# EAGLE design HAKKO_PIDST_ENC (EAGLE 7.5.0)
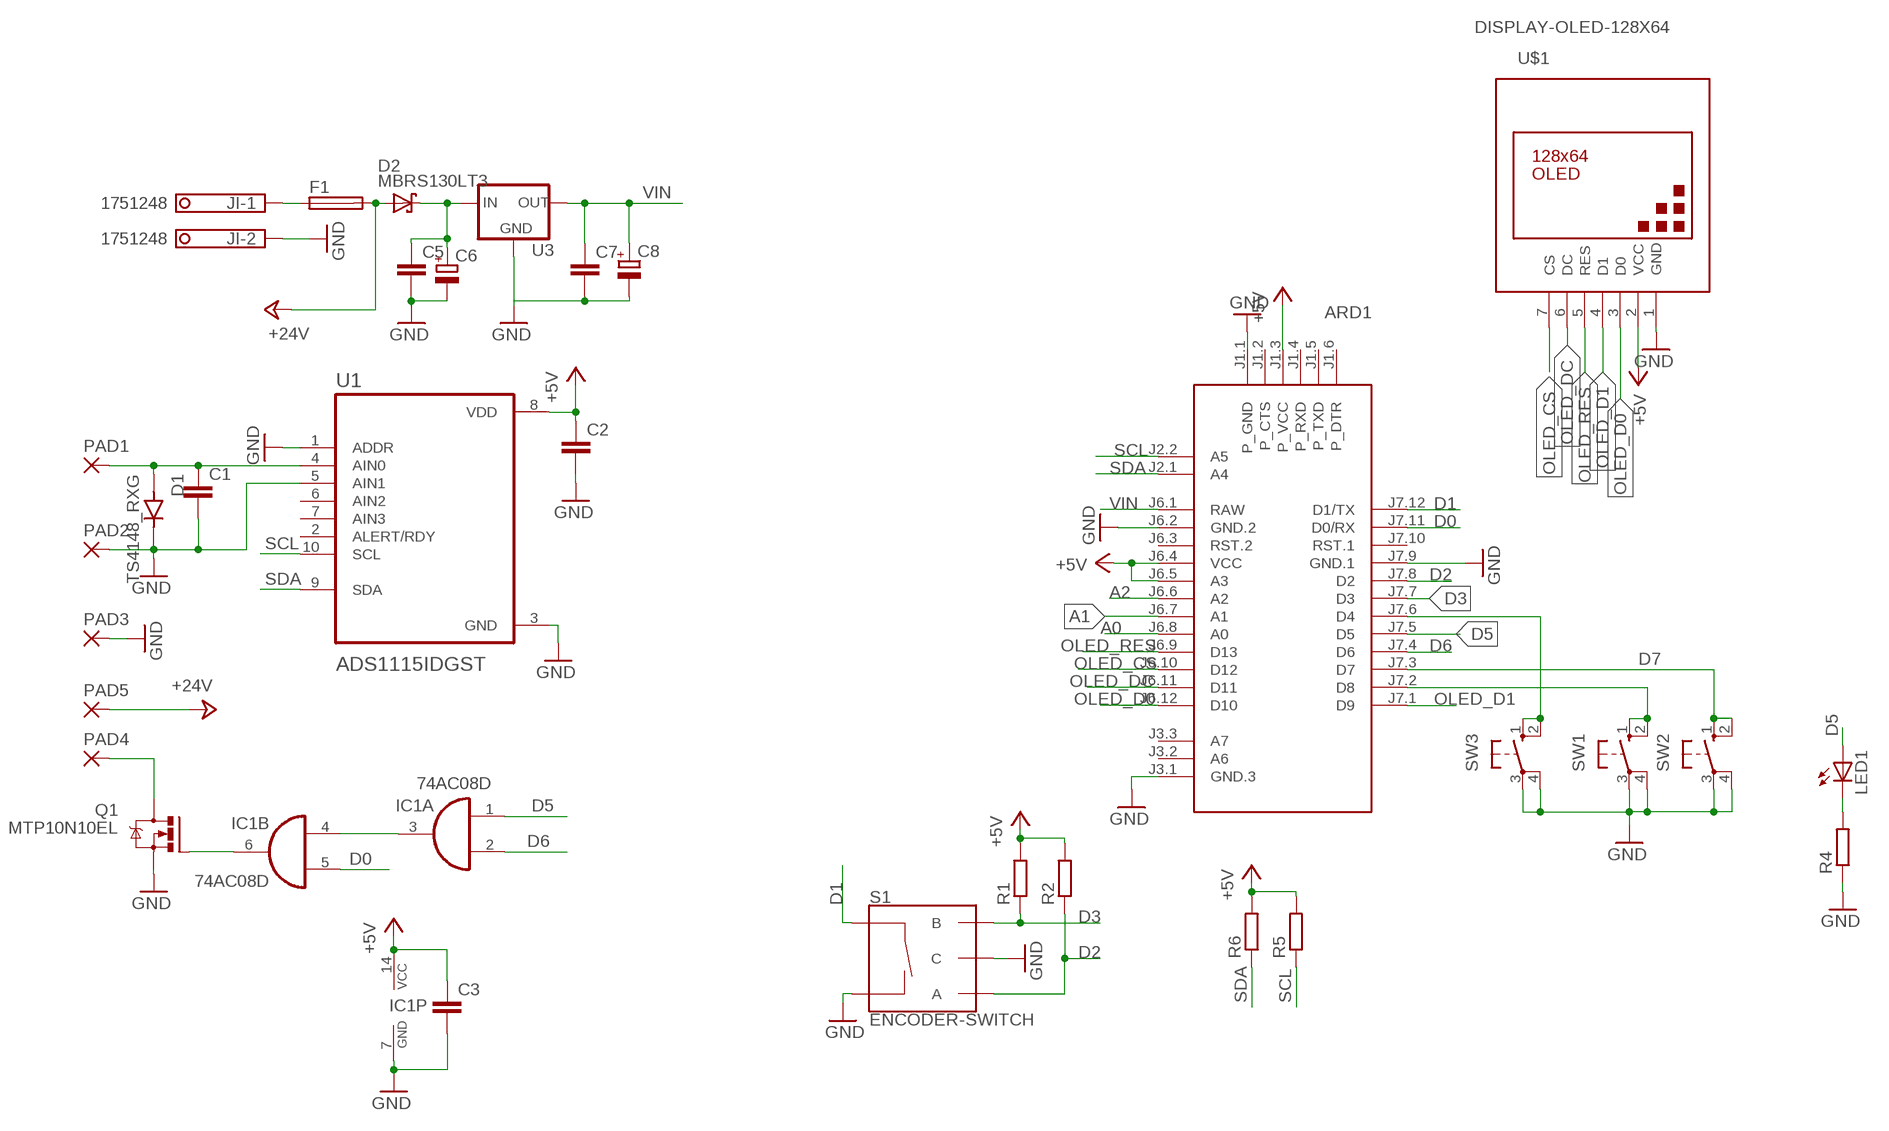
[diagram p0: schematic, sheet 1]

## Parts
ARD1  ARDUINO-PRO-MINI-3.3V  [ARDUINO-PRO-MINI]
C1  C-EUC1206  [C1206]
C2  C-EUC1206  [C1206]
C3  C-EUC1206  [C1206]
C5  C-EUC1206  [C1206]
C6  CPOL-EUSMCB  [SMC_B]
C7  C-EUC1206  [C1206]
C8  CPOL-EUSMCB  [SMC_B]
D1  TS4148_RXG  [DIO_TS4148_RXG]
D2  MBRS130LT3  [SMB]
F1  SH22,5  [SH22,5]
IC1  74AC08D  [SO14]
JI  1751248  [1751248]
LED1  LED5MM  [LED5MM]
PAD1  2,15/1,0  [2,15/1,0]
PAD2  2,15/1,0  [2,15/1,0]
PAD3  2,15/1,0  [2,15/1,0]
PAD4  2,15/1,0  [2,15/1,0]
PAD5  2,15/1,0  [2,15/1,0]
Q1  MTP10N10EL  IRLZ44Z  [TO220BH]
R1  R-EU_R1206  [R1206]
R2  R-EU_R1206  [R1206]
R4  R-EU_R1206  [R1206]
R5  R-EU_R1206  [R1206]
R6  R-EU_R1206  [R1206]
S1  ENCODER-SWITCH  [ROTARY_ENC_PLAIN]
SW1  10-XX  [B3F-10XX]
SW2  10-XX  [B3F-10XX]
SW3  10-XX  [B3F-10XX]
U1  ADS1115IDGST  [SOP50P490X110-10N]
U3  78LXX  [78LXX]
U$1  DISPLAY-OLED-128X64  [DISPLAY-OLED-128X64]

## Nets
+5V: ARD1.J1.3(P_VCC) ARD1.J6.4(VCC) ARD1.J6.5(A3) C2.1 C3.1 IC1.14(P:VCC) R1.2 R2.2 R5.2 R6.2 U1.8(VDD) U$1.2(VCC)
+24V: D2.A F1.2 PAD5.1(P)
A0: ARD1.J6.8(A0)
A1: ARD1.J6.7(A1)
A2: ARD1.J6.6(A2)
D0: ARD1.J7.11(D0/RX) IC1.5(B:I1)
D1: ARD1.J7.12(D1/TX) S1.SW+
D2: ARD1.J7.8(D2) R2.1 S1.A
D3: ARD1.J7.7(D3) R1.1 S1.B
D5: ARD1.J7.5(D5) IC1.1(A:I0) LED1.A
D6: ARD1.J7.4(D6) IC1.2(A:I1)
D7: ARD1.J7.3(D7) SW2.1(S) SW2.2(S1)
GND: ARD1.J1.1(P_GND) ARD1.J3.1(GND.3) ARD1.J6.2(GND.2) ARD1.J7.9(GND.1) C1.2 C2.2 C3.2 C5.2 C6.- C7.2 C8.- D1.C(K) IC1.7(P:GND) JI.2 PAD2.1(P) PAD3.1(P) Q1.S R4.1 S1.C S1.SW- SW1.3(P) SW1.4(P1) SW2.3(P) SW2.4(P1) SW3.3(P) SW3.4(P1) U1.1(ADDR) U1.3(GND) U1.5(AIN1) U3.GND U$1.1(GND)
N$1: C1.1 D1.A PAD1.1(P) U1.4(AIN0)
N$2: PAD4.1(P) Q1.D
N$3: IC1.3(A:O) IC1.4(B:I0)
N$4: F1.1 JI.1
N$6: C5.1 C6.+ D2.C U3.IN
N$7: LED1.K(C) R4.2
N$8: ARD1.J7.2(D8) SW1.1(S) SW1.2(S1)
N$9: IC1.6(B:O) Q1.G
N$10: ARD1.J7.6(D4) SW3.1(S) SW3.2(S1)
OLED_CS: ARD1.J6.10(D12) U$1.7(CS)
OLED_D0: ARD1.J6.12(D10) U$1.3(D0)
OLED_D1: ARD1.J7.1(D9) U$1.4(D1)
OLED_DC: ARD1.J6.11(D11) U$1.6(DC)
OLED_RES: ARD1.J6.9(D13) U$1.5(RES)
SCL: ARD1.J2.2(A5) R5.1 U1.10(SCL)
SDA: ARD1.J2.1(A4) R6.1 U1.9(SDA)
VIN: ARD1.J6.1(RAW) C7.1 C8.+ U3.OUT
Unconnected: ARD1.J1.2(P_CTS) ARD1.J1.4(P_RXD) ARD1.J1.5(P_TXD) ARD1.J1.6(P_DTR) ARD1.J3.2(A6) ARD1.J3.3(A7) ARD1.J6.3(RST.2) ARD1.J7.10(RST.1) IC1.8(C:O) IC1.9(C:I0) IC1.10(C:I1) IC1.11(D:O) IC1.12(D:I0) IC1.13(D:I1) U1.2(ALERT/RDY) U1.6(AIN2) U1.7(AIN3)

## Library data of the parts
ARD1 = diy-modules:ARDUINO-PRO-MINI-*: Arduino Pro Mini and compatible devices More details available here: https://www.arduino.cc/en/Main/ArduinoBoardProMini Click here to find device on ebay.com
C1-C3 C5 C7 = rcl:C-EU: CAPACITOR, European symbol
C6 C8 = rcl:CPOL-EU: POLARIZED CAPACITOR, European symbol
D1 = TS4148_RXG:TS4148_RXG: Check availability Check availability Check availability; AVAILABILITY: In Stock; CHECK_PRICES: https://www.snapeda.com/parts/TS4148%20RXG/Taiwan+Semiconductor/view-part/?ref=eda; DESCRIPTION: 1206 (Ceramics) 75V 0.15A Switching Diode & Array; MF: Taiwan Semiconductor; MP: TS4148 RXG; PACKAGE: 1206-2 Taiwan Semiconductor; PRICE: None; SNAPEDA_LINK: https://www.snapeda.com/parts/TS4148%20RXG/Taiwan+Semiconductor/view-part/?ref=snap
D2 = diode:MBRS130LT3: Schottky Power Rectifier
F1 = fuse:SH22,5: FUSE HOLDER; MF: SCHURTER; MPN: 0031.8201; OC_FARNELL: 1162740; OC_NEWARK: 96F8317
IC1 = 74xx-eu:74*08: Quad 2-input AND gate
JI = con-phoenix-350:1751248: MKDS 1/ 2-3,5 Printklemme; OC_FARNELL: unknown; OC_NEWARK: unknown
LED1 = led:LED: LED
PAD1-PAD5 = wirepad:2,15/1,0: THROUGH-HOLE PAD
Q1 = transistor-power:IRLZ44Z: N-Channel HEXFET® Power MOSFET Logic Level AUTOMOTIVE MOSFET Source: http://www.irf.com/product-info/datasheets/data/irlz44zpbf.pdf
R1 R2 R4-R6 = rcl:R-EU_: RESISTOR, European symbol
S1 = SparkFun-Switches:ENCODER-SWITCH: Rotary Encoder w/ Select Switch Encoders rotate similarly to potentiometers, but they’re different from potentiometers in that an encoder has full rotation without limits. They output gray code so that you can tell how much and in which direction the encoder has been turned. This encoder includes a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; SF_SKU: COM-09117
SW1-SW3 = switch-omron:10-XX: OMRON SWITCH; MPN: B3F-1000; OC_FARNELL: 176432; OC_NEWARK: 36M3542
U1 = ADS1115IDGST:ADS1115IDGST: Check availability; AVAILABILITY: In Stock; CHECK_PRICES: https://www.snapeda.com/parts/ADS1115IDGST/Texas+Instruments/view-part/?ref=eda; DESCRIPTION: 16-bit, 860-SPS, 4-channel, delta-sigma ADC with PGA, oscillator, VREF, comparator and I2C; MF: Texas Instruments; MP: ADS1115IDGST; PACKAGE: VSSOP-10 Texas Instruments; PRICE: None; SNAPEDA_LINK: https://www.snapeda.com/parts/ADS1115IDGST/Texas+Instruments/view-part/?ref=snap
U3 = v-reg:78LXX: VOLTAGE REGULATOR
U$1 = diy-modules:DISPLAY-OLED-128X64: 128x64 Dot Matrix OLED Module based on SSD1306 chip Variant with SPI interface More details available here: http://www.instructables.com/id/How-to-use-OLED-display-arduino-module/ SSD1306 datasheet: https://cdn-shop.adafruit.com/datasheets/SSD1306.pdf Click here to find device on ebay.com Note: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

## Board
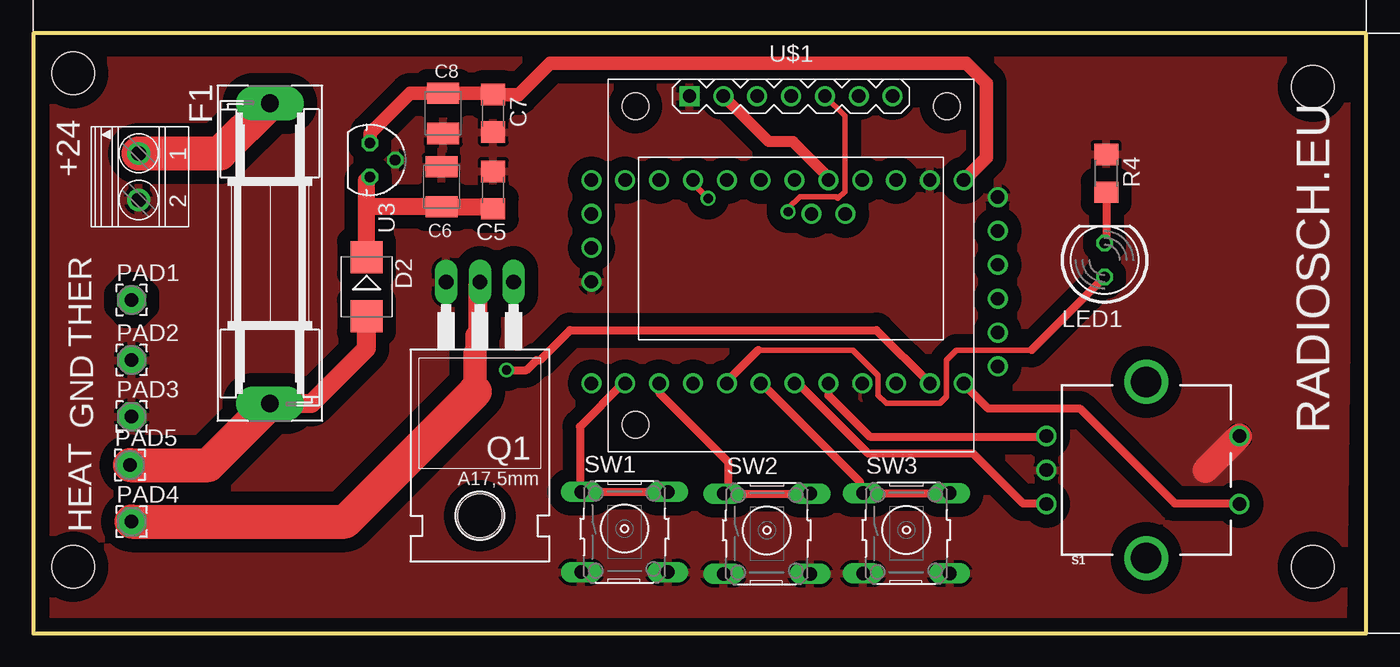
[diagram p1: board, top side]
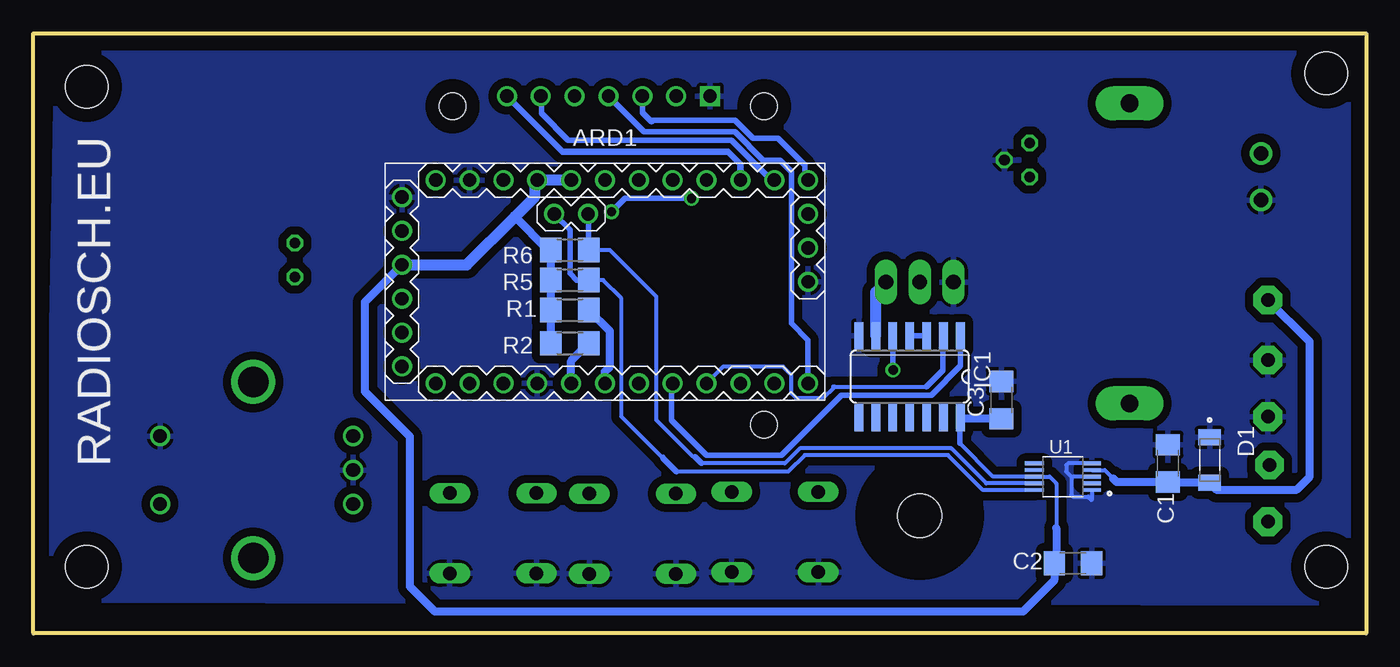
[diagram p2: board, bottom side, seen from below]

Size 100 x 45 mm. Coordinates in mm from the lower left corner, seen from the top.
Outline: 0,0 100,0 100,45 0,45 0,0
Copper layers (1*16): Top 0.035mm / dielectric 1.5mm / Bottom 0.035mm
Design rules "default *": minimum track width 10mil, minimum drill 24mil, track to track 6mil, track to pad 8mil, pad to pad 8mil, via to via 8mil, smd to smd 8mil, copper to edge 40mil, drill to drill 8mil, minimum pad ring 8mil, minimum via ring 8mil, stop-mask expansion 4mil, vias tented up to drill 0mil, thermal gap 10mil
Holes 3.2 mm at 3,42 3,5 96,5 96,41

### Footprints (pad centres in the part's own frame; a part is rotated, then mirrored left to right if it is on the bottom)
ARDUINO-PRO-MINI = drill 1: J1.1 -15.24,6.35; J1.2 -15.24,3.81; J1.3 -15.24,1.27; J1.4 -15.24,-1.27; J1.5 -15.24,-3.81; J1.6 -15.24,-6.35; J2.1 -1.27,5.08; J2.2 -3.81,5.08; J3.1 15.24,0; J3.2 15.24,2.54; J3.3 15.24,5.08; J6.1 -12.7,7.62; J6.2 -10.16,7.62; J6.3 -7.62,7.62; J6.4 -5.08,7.62; J6.5 -2.54,7.62; J6.6 0,7.62; J6.7 2.54,7.62; J6.8 5.08,7.62; J6.9 7.62,7.62; J6.10 10.16,7.62; J6.11 12.7,7.62; J6.12 15.24,7.62; J7.1 15.24,-7.62; J7.2 12.7,-7.62; J7.3 10.16,-7.62; J7.4 7.62,-7.62; J7.5 5.08,-7.62; J7.6 2.54,-7.62; J7.7 0,-7.62; J7.8 -2.54,-7.62; J7.9 -5.08,-7.62; J7.10 -7.62,-7.62; J7.11 -10.16,-7.62; J7.12 -12.7,-7.62
C1206 = smd 1.6 x 1.8: 1 -1.4,0; 2 1.4,0
SMC_B = smd 1.6 x 2.4: + -1.5,0; - 1.5,0
DIO_TS4148_RXG = smd 1.2 x 1.7: A 1.7,0; C -1.7,0
SMB = smd 2.4 x 2.4: A 2.2,0; C -2.2,0
SH22,5 = drill 1.321 pad 2.54 long: 1 -11.252,0; 2 11.252,0
SO14 = smd 0.66 x 2.032: 1 -3.81,-3.073; 2 -2.54,-3.073; 3 -1.27,-3.073; 4 0,-3.073; 5 1.27,-3.073; 6 2.54,-3.073; 7 3.81,-3.073; 8 3.81,3.073; 9 2.54,3.073; 10 1.27,3.073; 11 0,3.073; 12 -1.27,3.073; 13 -2.54,3.073; 14 -3.81,3.073
1751248 = drill 1.1 pad 1.7: 1 -1.75,-0.1; 2 1.75,-0.1
LED5MM = drill 0.813 octagon: A -1.27,0; K 1.27,0
2,15/1,0 = drill 1.016 pad 2.159 octagon: 1 0,0
TO220BH = drill 1.118 long: D 0,-6.35; G -2.54,-6.35; S 2.54,-6.35 | hole 3.302: 0,11.176
R1206 = smd 1.6 x 1.803: 1 -1.422,0; 2 1.422,0
ROTARY_ENC_PLAIN = drill 1.016: A 7.493,-2.54; B 7.493,2.54; C 7.493,0; SW+ -6.985,2.54; SW- -6.985,-2.54 | drill 2.286: P$3 0,6.604; P$4 0,-6.604
B3F-10XX = drill 1.016 long: 1 -3.251,2.761; 2 3.251,2.761; 3 -3.251,-3.261; 4 3.251,-3.261
SOP50P490X110-10N = smd 1.47 x 0.28: 1 -2.15,1; 2 -2.15,0.5; 3 -2.15,0; 4 -2.15,-0.5; 5 -2.15,-1; 6 2.15,-1; 7 2.15,-0.5; 8 2.15,0; 9 2.15,0.5; 10 2.15,1
78LXX = drill 0.813 octagon: GND 0,1.905; IN 1.27,0; OUT -1.27,0
DISPLAY-OLED-128X64 = drill 1 square: 1 -7.62,12.7 | drill 1: 2 -5.08,12.7; 3 -2.54,12.7; 4 0,12.7; 5 2.54,12.7; 6 5.08,12.7; 7 7.62,12.7 | hole 2: -11.684,11.938; 11.684,11.938; -11.684,-11.938

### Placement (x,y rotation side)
ARD1  57.11,26.37 0 bottom
C1  14.88,12.75 90 bottom
C2  22,5.25 0 bottom
C3  27.38,17.5 90 bottom
C5  34.5,33.25 90 top
C6  30.62,33.5 90 top
C7  34.5,39 270 top
C8  30.75,39 270 top
D1  11.75,13 270 bottom
D2  25,26 270 top
F1  17.75,28.5 270 top
IC1  34.25,19.25 180 bottom
JI  8,34.25 270 top
LED1  80.38,28 90 top
PAD1  7.38,25 0 top
PAD2  7.38,20.5 0 top
PAD3  7.38,16.25 0 top
PAD4  7.38,8.38 0 top
PAD5  7.25,12.62 0 top
Q1  33.5,20 180 top
R1  59.75,24.25 180 bottom
R2  59.75,21.75 180 bottom
R4  80.5,34.5 270 top
R5  59.75,26.5 180 bottom
R6  59.75,28.75 180 bottom
S1  83.5,12.25 180 top
SW1  44.35,7.85 0 top
SW2  55.03,7.72 0 top
SW3  65.5,7.75 0 top
U1  22.75,11.75 180 bottom
U3  25.25,35.5 270 top
U$1  56.85,27.59 0 top

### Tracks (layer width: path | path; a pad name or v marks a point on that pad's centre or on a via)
+5V
  Top 0.813: ARD1.J6.5 59.65,34.23 57,36.88 55.19,36.88 U$1.2
  Bottom 0.305: 23.25,7.9 23.25,11.25 23.75,11.75 U1.8 28,11.75 30.5,14.25
  Bottom 0.406: 30.5,14.25 30.5,16.12 IC1.14
  Bottom 0.61: ARD1.J1.3 75.12,24.86 75.12,18.12 71.75,14.75 71.75,3.5 69.88,1.62 25.75,1.62 23.4,3.98 C2.1 23.25,5.4 23.25,7.9 | R2.2 R1.2 R5.2 R6.2 61.38,28.75 63.88,31.25 | C3.1 30.36,16.1 IC1.14
  Bottom 0.813: ARD1.J6.5 ARD1.J6.4 62.38,33.8 62.38,32.75 63.88,31.25 67.48,27.64 ARD1.J1.3
+24V
  Top 1.422: F1.2 20.87,17.25 25,21.38 D2.A
  Top 2.54: PAD5.1 13.13,12.62 F1.2
D0  (via drill 0.7)
  Top 0.61: v35.5,19.75 37,19.75 37.75,20.5 38,20.5 40.25,22.75 63.27,22.75 ARD1.J7.11
  Bottom 0.406: IC1.5 35.52,19.77 v35.5,19.75
D1
  Top 0.61: ARD1.J7.12 69.81,18.69 71.62,16.88 78.5,16.88 85.62,9.75 90.44,9.75 S1.SW+
D2
  Top 0.61: ARD1.J7.8 59.65,17.85 62.75,14.75 75.97,14.75 S1.A
  Bottom 0.61: ARD1.J7.8 59.65,20.43 R2.1
D3
  Top 0.61: ARD1.J7.7 57.38,18.75 62.62,13.5 70.5,13.5 74.25,9.75 75.97,9.75 S1.B
  Bottom 0.61: ARD1.J7.7 57.11,19.64 56.75,20 56.75,22.67 R1.1
D5
  Top 0.406: 74.89,21.25 69.25,21.25 68.5,20.5 68.5,17.75 68,17.25 64,17.25 63.38,17.88 63.38,19.38 61.5,21.25 54.38,21.25
  Top 0.61: ARD1.J7.5 52.03,18.91 54.38,21.25 | 74.89,21.25 LED1.A
  Bottom 0.406: IC1.1 30.44,20.06 32.62,17.88 39.38,17.88 43.88,13.38 49.5,13.38 52.12,16 52.12,18.66 ARD1.J7.5
D6
  Bottom 0.305: 40,18.5 39.88,18.5 | 39.88,18.5 33,18.5 | 49.49,18.62 ARD1.J7.4 48.24,20 43.75,20 43.12,19.38 43.12,18 42.75,17.62 40.75,17.62 39.88,18.5
  Bottom 0.406: 33,18.5 31.75,19.75 31.75,22.28 IC1.2
D7
  Top 0.61: SW2.2 SW2.1 52.12,10.83 52.12,12.88 46.95,18.05 ARD1.J7.3
GND
  Top 1.93: 87.94,12.25 S1.SW-
  Bottom 0.305: U1.1 20.6,10.03 20.62,10 20.88,10.25 22,10.25 22.12,10.38 22.12,11.75 | U1.3 22.12,11.75 | U1.5 22.38,12.75 22.5,12.62 22.5,12.12 22.12,11.75
  pour Top (isolate 1.016): 1,43 98.75,43 98.25,0.5 1.5,0.5
  pour Bottom (isolate 0.61): 1.25,43.5 98.25,43.5 99,2.5 0.5,2.25
N$1
  Bottom 0.305: U1.4 19.62,12.25 19,11.62
  Bottom 0.61: PAD1.1 4.25,21.88 4.25,11.75 5.25,10.75 11.2,10.75 D1.A 14.82,11.3 C1.1 18.73,11.35 19,11.62
N$2
  Top 1.422: 33.12,21 33.12,22.38 33.38,22.62 33.38,26.23 Q1.D
  Top 1.778: 33.12,18.12 33.12,21
  Top 2.54: PAD4.1 23.38,8.38 33.12,18.12
N$3
  Bottom 0.406: IC1.4 IC1.3
N$4
  Top 2.54: JI.1 14,36 F1.1
N$6
  Top 1.27: D2.C 25,32.25 | 25,32.25 25,33.98 U3.IN | 25,32.25 25.25,32 C6.+ 34.35,32 C5.1
N$7
  Top 0.61: R4.2 80.5,29.39 LED1.K
N$8
  Top 0.61: ARD1.J7.2 44.25,18.75 41,15.5 41,10.71 SW1.1 SW1.2
N$9
  Bottom 0.813: IC1.6 36.79,25.6 Q1.G
N$10
  Top 0.61: ARD1.J7.6 54.62,18.75 62,11.38 62,10.76 SW3.1 SW3.2
OLED_CS
  Bottom 0.5: ARD1.J6.10 46.95,35.2 47.88,36.12 60.3,36.12 U$1.7
OLED_D0
  Bottom 0.406: U$1.3 54.31,39.06 53.62,38.38 53.5,38.5 47.38,38.5 46,37.12 44.12,37.12 42.12,35.12 42.12,34.25 ARD1.J6.12
OLED_D1
  Bottom 0.406: ARD1.J7.1 41.87,21.99 43.12,23.25 43.12,34.62 44,35.5 45.25,35.5 47.38,37.62 54.19,37.62 U$1.4
OLED_DC
  Bottom 0.406: ARD1.J6.11 44.62,33.99 47.62,37 59.88,37 61.88,39 61.88,40.23 U$1.6
OLED_RES  (via drill 0.7)
  Top 0.406: U$1.5 60.88,38.8 60.88,33.12 60.38,32.62 60.25,32.75 57.5,32.75 56.62,31.88 v56.62,31.62
  Top 0.5: ARD1.J6.9 49.49,33.76 v50.62,32.62
  Bottom 0.406: v50.62,32.62 55.62,32.62 v56.62,31.62
SCL
  Bottom 0.305: 52.81,13.19 55.88,16.25 55.88,25.12 57.25,26.5 R5.1 | 52.75,13.25 52.81,13.19 | 52.12,12.5 52.75,13.12 52.81,13.19 | U1.10 28.75,10.75 31.38,13.38 42.12,13.38 43.38,12.12 51.75,12.12
  Bottom 0.406: R5.1 59.25,26.5 59.75,27 59.75,30.28 ARD1.J2.2 | 51.75,12.12 52.75,13.12
SDA
  Bottom 0.305: 50.38,13.25 50.5,13.25 53.25,16 53.25,25.25 56.75,28.75 R6.1 | 49.88,12.75 43.62,12.75 42.5,13.88 31.12,13.88 28.5,11.25 U1.9
  Bottom 0.406: R6.1 58.33,31.4 ARD1.J2.1 | 49.88,12.75 50.38,13.25
VIN
  Top 1.016: U3.OUT 25.25,37.5 28.25,40.5 C8.+ 34.4,40.5 C7.1 36.4,40.4 38.75,42.75 70,42.75 71.5,41.25 71.5,35.68 ARD1.J6.1

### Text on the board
tPlace: +24 | THER | GND | RADIOSCH.EU | HEAT
bPlace: RADIOSCH.EU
